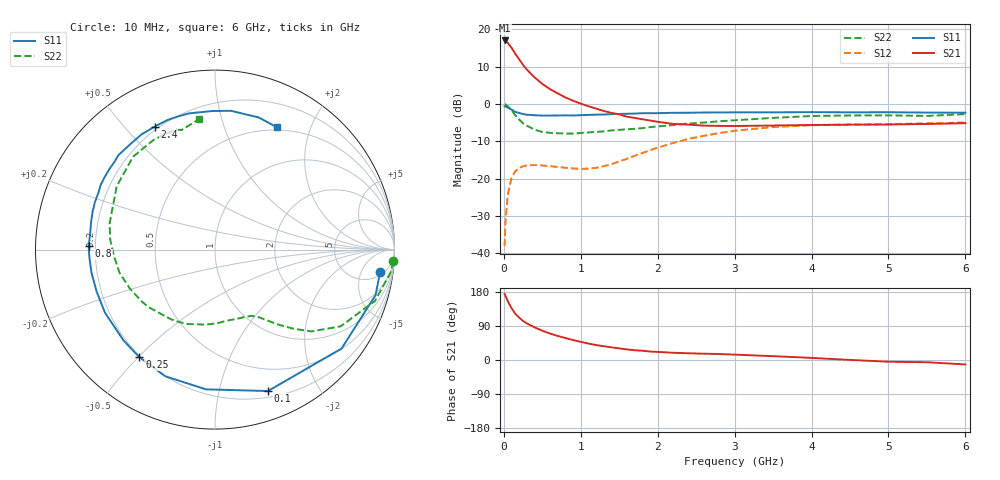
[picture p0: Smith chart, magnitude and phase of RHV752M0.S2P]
! SIEMENS Small Signal Semiconductors
! BFR106
! Si NPN RF Bipolar Junction Transistor in SOT23
! VCE = 0.75 V  IC = 2 mA
! Common Emitter S-Parameters:  August  1996
# GHz  S  MA  R  50
!  f  S11  S21  S12  S22
! GHz  MAG  ANG  MAG  ANG  MAG  ANG  MAG  ANG
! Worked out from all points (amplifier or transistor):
!   36 points, 10 MHz to 6 GHz, reference 50 ohm
!   highest |S21| = 17.0 dB at 10 MHz (marker M1)
!   |S21| within 3 dB of that: start of sweep to 131.9 MHz
!   unconditionally stable (mu >= 1): 755 MHz to end of sweep
!   at 250 MHz: K = 0.34, MSG = 13.6 dB, |S12| = -16.7 dB
!   at 1.4 GHz: K = 1.37, MAG = 3.2 dB, |S12| = -16.1 dB
!   at 6 GHz: K = 1.03, MAG = -1.1 dB, |S12| = -5.0 dB
!   S11 on the Smith chart (normalised r, x): 10 MHz: 6, -11; 100 MHz: 0.26, -1.41; 250 MHz: 0.19, -0.50; 800 MHz: 0.17, +0.01; 2.4 GHz: 0.19, +0.61; 6 GHz: 0.47, +1.52
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0.01  0.9281 -7.8  7.08 174.3  0.0125 87.1  0.9962 -3.8
0.02  0.93 -15.8  7.025 170.2  0.0251 81.8  0.9863 -7.5
0.05  0.8952 -38.0  6.595 155.6  0.0601 68.6  0.9361 -17.8
0.1  0.8414 -69.5  5.656 137.0  0.1026 52.7  0.8203 -31.4
0.15  0.7802 -93.7  4.679 121.8  0.1263 40.5  0.7048 -40.3
0.2  0.7581 -111.4  3.95 111.6  0.1394 33.3  0.6184 -45.4
0.25  0.7326 -125.1  3.333 102.8  0.1468 27.4  0.5512 -49.5
0.3  0.7185 -135.1  2.876 96.5  0.1507 24.1  0.5114 -52.1
0.4  0.7067 -150.1  2.266 86.1  0.152 19.2  0.4522 -56.7
0.5  0.6997 -160.5  1.854 77.3  0.1503 16.8  0.4224 -60.9
0.6  0.7001 -169.4  1.582 69.9  0.1473 16.1  0.4109 -65.6
0.8  0.7041 178.5  1.225 58.0  0.1401 18.5  0.4018 -76.1
1.1  0.714 162.7  0.932 43.4  0.1363 29.9  0.4158 -93.2
1.6  0.7397 142.8  0.676 27.9  0.1848 49.1  0.459 -122.0
2.2  0.7615 122.5  0.541 19.1  0.3005 49.2  0.522 -155.5
2.4  0.7631 116.2  0.529 17.7  0.3402 46.1  0.5475 -166.4
3  0.7725 100.7  0.507 14.2  0.4379 33.9  0.6051 166.0
3.5  0.7725 90.9  0.515 10.1  0.4909 23.6  0.6515 147.2
4.5  0.7726 77.3  0.529 0.2  0.5301 6.3  0.7013 118.8
5  0.7756 71.8  0.531 -4.6  0.5354 -0.1  0.7041 108.4
5.5  0.767 66.9  0.54 -5.9  0.5502 -3.3  0.6919 105.6
6  0.7635 63.2  0.553 -11.7  0.5641 -9.9  0.7313 97.0
